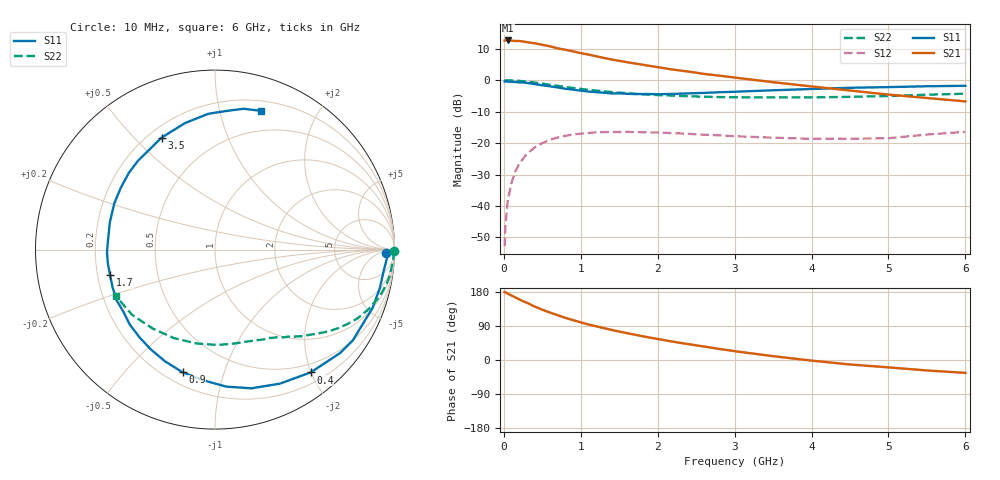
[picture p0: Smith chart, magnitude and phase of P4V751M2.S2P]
! SIEMENS Small Signal Semiconductors
! BFP182
! Si NPN RF Bipolar Junction Transistor in SOT143
! VCE = 0.75 V  IC = 1.2 mA
! Common Emitter S-Parameters:  March  1996
# GHz  S  MA  R  50
!  f  S11  S21  S12  S22
! GHz  MAG  ANG  MAG  ANG  MAG  ANG  MAG  ANG
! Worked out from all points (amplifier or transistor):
!   36 points, 10 MHz to 6 GHz, reference 50 ohm
!   highest |S21| = 12.6 dB at 50 MHz (marker M1)
!   |S21| within 3 dB of that: start of sweep to 806.8 MHz
!   unconditionally stable (mu >= 1): 2.412 GHz to end of sweep
!   at 250 MHz: K = 0.11, MSG = 18.6 dB, |S12| = -25.0 dB
!   at 1.4 GHz: K = 0.60, MSG = 11.5 dB, |S12| = -16.5 dB
!   at 6 GHz: K = 1.27, MAG = 1.7 dB, |S12| = -16.4 dB
!   S11 on the Smith chart (normalised r, x): 10 MHz: 34, -15; 400 MHz: 0.36, -1.99; 900 MHz: 0.27, -0.73; 1.7 GHz: 0.25, -0.11; 3.5 GHz: 0.25, +0.60; 6 GHz: 0.29, +1.34
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0.01  0.9521 -1.2  4.266 179.4  0.0023 85.7  0.997 -0.5
0.02  0.9594 -2.8  4.277 178.7  0.0047 94.5  0.9945 -1.1
0.05  0.9477 -7.0  4.28 175.0  0.0121 87.6  0.9955 -2.9
0.1  0.943 -13.3  4.244 170.1  0.0236 81.0  0.9889 -5.7
0.15  0.9359 -20.4  4.192 165.1  0.0356 77.3  0.9838 -8.6
0.2  0.9213 -27.1  4.198 159.9  0.0466 73.6  0.9752 -11.3
0.25  0.9197 -33.3  4.111 155.2  0.0565 69.5  0.9617 -14.1
0.4  0.8673 -52.1  3.859 141.2  0.0852 58.3  0.9174 -21.3
0.5  0.8299 -64.1  3.648 132.7  0.1 51.3  0.8822 -25.7
0.6  0.7991 -75.3  3.457 125.1  0.1129 45.4  0.8458 -29.4
0.8  0.7306 -95.3  3.042 111.2  0.1305 35.1  0.7821 -35.5
0.9  0.7069 -104.8  2.871 105.2  0.137 30.8  0.7528 -38.0
1.1  0.6604 -123.1  2.554 93.7  0.1451 22.9  0.7027 -42.7
1.4  0.6168 -145.7  2.133 79.6  0.1501 13.6  0.6492 -48.5
1.7  0.6017 -166.5  1.843 66.9  0.1497 7.0  0.6085 -53.3
1.9  0.6019 -178.5  1.685 59.1  0.1477 3.5  0.588 -56.7
2.2  0.6054 165.3  1.473 48.3  0.144 -0.7  0.569 -61.6
2.8  0.6427 138.3  1.18 29.2  0.1328 -5.6  0.5388 -72.8
3.5  0.6913 115.5  0.929 10.1  0.1219 -6.7  0.5317 -88.5
4.5  0.7575 92.9  0.685 -11.8  0.1171 -1.0  0.5437 -115.0
5.5  0.8007 78.5  0.521 -27.6  0.1368 6.0  0.5879 -141.8
6  0.8144 71.7  0.46 -34.0  0.1509 5.0  0.6094 -154.7
